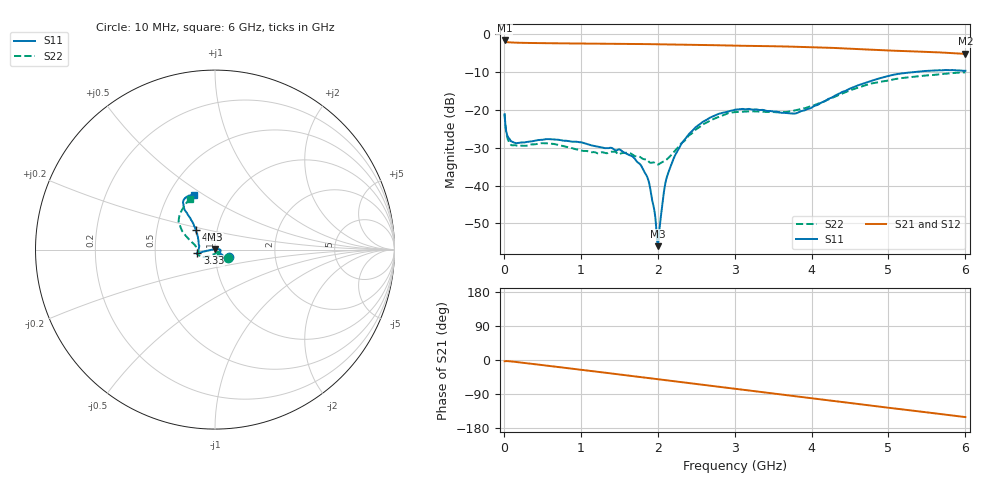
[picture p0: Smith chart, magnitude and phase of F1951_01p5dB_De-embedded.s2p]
! Integrated Device Technology
! Corporate Headquarters
! 6024 Silver Creek Valley Road
! San Jose, CA 95138  USA
! Phone:  1-408-284-8200
! Toll Free:  1-800-223-1366
! Webpage:  http://www.idt.com/
! Timing and RF Division
! 515 Groton Road, Suite 102
! Westford, MA 01886-6024
! Device:  F1951
! Description: 6-bit 0.5 dB Digital Step Attenuator
! Frequency:  100.0 -  4000.00 MHz
! Package:  4x4 mm Thin QFN Plastic Package: 24 pin
! Ports:  2 RF, 6 DC
!  Pin  1  = NC
!  Pin  2  = RF1  =  Port 1
!  Pin  3  = GND
!  Pin  4  = NC
!  Pin  5  = Serial Data Out (SDO)
!  Pin  6  = NC
!  Pin  7  = Reset Bar ( RSTb)
!  Pin  8  = Clock (CLK)
!  Pin  9  = Chip Select Bar (CSb)
!  Pin 10  = NC
!  Pin 11  = Serial Data In (SDI)
!  Pin 12  = NC
!  Pin 13  = NC
!  Pin 14  = VDD
!  Pin 15  = NC
!  Pin 16  = GND
!  Pin 17  = RF2  =  Port 2
!  Pin 18  = NC
!  Pin 19  = GND
!  Pin 20  = GND
!  Pin 21  = GND
!  Pin 22  = GND
!  Pin 23  = GND
!  Pin 24  = GND
! State:  3
! Atten State:  1.5 dB
! Voltage:  +3.30 Volts
! Current:  0.488 mA
! Data:  The device was measured on a F195X evaluation board which has
!  individual transmission lines to the RF pins.  Data was collected
!  de-embedded using a Automatic Fixture Removal [AFR] (Keysight Technologies).
!  The reference plane is the edge of the package pin.
! Misc:  Lot Code  1225BCA
!  Action Tracker AT0399
! Date Measured:  2018-09-13
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# GHz S dB R 50
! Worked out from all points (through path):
!   600 points, 10 MHz to 6 GHz, reference 50 ohm
!   highest |S21| = -1.70 dB at 10 MHz (marker M1); lowest = -5.2 dB at 6 GHz (marker M2)
!   group delay of S21, straight-line fit = 69.5 ps
!   lowest |S11| = -56.0 dB at 2 GHz (marker M3), VSWR 1.00, Z = 50 + j0.155 ohm
!   |S11| at or under -10 dB: start of sweep to 5.35 GHz
!   |S22| runs from -34.4 to -10.1 dB; largest |S21 - S12| = 0.00091
!   S11 on the Smith chart (normalised r, x): 10 MHz: 1.16, -0.10; 3.33 GHz: 0.82, -0.03; 4.29 GHz: 0.79, +0.17; 6 GHz: 0.66, +0.45
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0.01  -21.15 -30.0  -1.70 -3.3  -1.70 -3.3  -21.22 -32.5
0.06  -27.39 -35.8  -2.19 -3.1  -2.19 -3.1  -28.17 -40.2
0.11  -28.45 -40.6  -2.24 -4.0  -2.25 -4.0  -29.37 -44.3
0.61  -27.77 -61.5  -2.43 -16.1  -2.43 -16.1  -28.94 -66.1
1.01  -28.60 -40.6  -2.51 -26.0  -2.52 -26.0  -30.76 -45.4
1.51  -30.51 -3.1  -2.60 -38.2  -2.60 -38.2  -31.60 -9.1
1.77  -34.35 7.6  -2.64 -44.8  -2.64 -44.8  -32.44 -18.1
1.88  -38.68 9.8  -2.67 -47.6  -2.67 -47.6  -33.60 -31.4
2  -55.99 102.8  -2.69 -50.6  -2.70 -50.6  -34.44 -58.9
2.01  -54.71 138.6  -2.70 -50.9  -2.70 -50.9  -34.43 -62.0
2.03  -50.11 165.4  -2.70 -51.4  -2.70 -51.4  -34.17 -68.0
2.08  -41.82 174.9  -2.72 -52.7  -2.72 -52.7  -33.60 -78.7
2.12  -37.69 -178.9  -2.73 -53.7  -2.73 -53.7  -33.07 -89.4
2.31  -28.93 -172.5  -2.78 -58.5  -2.79 -58.6  -28.81 -121.3
2.6  -23.01 -169.7  -2.89 -66.0  -2.89 -66.0  -23.73 -141.9
3.01  -19.96 -167.0  -3.06 -76.2  -3.06 -76.2  -20.61 -156.9
3.33  -20.06 -169.8  -3.17 -84.1  -3.17 -84.1  -20.50 -165.9
3.77  -20.99 168.3  -3.35 -95.3  -3.35 -95.3  -20.22 178.7
4.01  -19.32 148.9  -3.47 -101.4  -3.47 -101.4  -18.98 168.8
4.29  -16.45 134.5  -3.67 -108.5  -3.67 -108.5  -16.66 160.0
5.01  -11.02 127.3  -4.36 -126.2  -4.36 -126.2  -12.23 144.4
6  -9.71 111.4  -5.23 -150.6  -5.23 -150.6  -10.09 116.2
